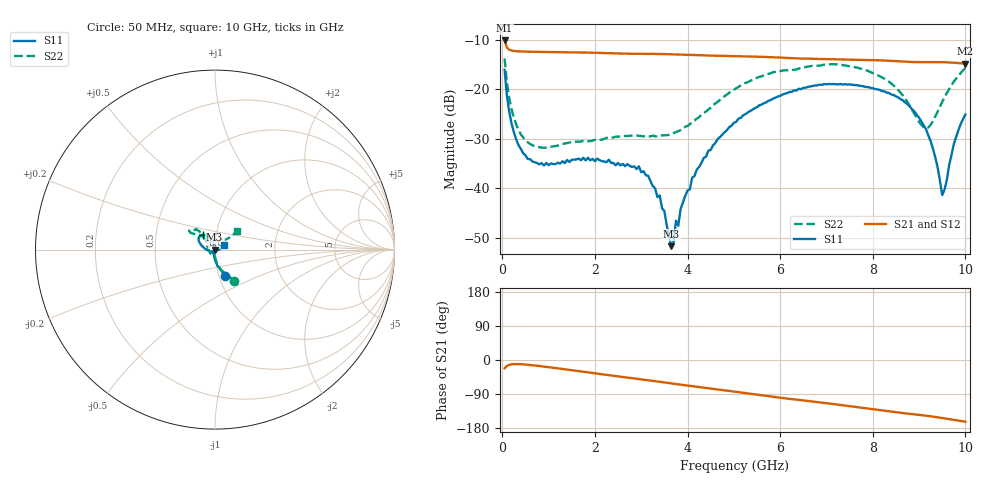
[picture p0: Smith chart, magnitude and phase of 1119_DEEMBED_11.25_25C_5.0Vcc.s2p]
!Hittite Microwave Corp.
!Digital Attenuator/PhaseShifter Rev 1.4.0
!Filename: C:\DATA\DATA\1119_DEEMBED_11.25_25C_5.0Vcc.s2p
!VNA ID: Agilent Technologies,N5224A,MY51441122,A.10.45.03
!Device type:
!2 Port Calibration.
!Temp(C): 25
!Lot Number:
!Serial Number:
!Operator:
!Misc:
!Attenuator:  11.250
# GHZ S DB R 50.0
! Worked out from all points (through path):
!   200 points, 50 MHz to 10 GHz, reference 50 ohm
!   highest |S21| = -10.14 dB at 50 MHz (marker M1); lowest = -14.8 dB at 10 GHz (marker M2)
!   group delay of S21, straight-line fit = 43.4 ps
!   lowest |S11| = -51.7 dB at 3.65 GHz (marker M3), VSWR 1.01, Z = 49.7 + j0.0195 ohm
!   |S11| at or under -10 dB: start of sweep to end of sweep
!   |S22| runs from -31.8 to -13.8 dB; largest |S21 - S12| = 0.00059
!   S11 on the Smith chart (normalised r, x): 50 MHz: 1.07, -0.32; 6.6 GHz: 0.86, +0.14; 10 GHz: 1.10, +0.06
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0.05  -16.07 -69.0  -10.14 -21.6  -10.14 -21.6  -13.79 -58.5
0.1  -21.37 -82.7  -11.60 -15.9  -11.59 -15.9  -18.60 -73.4
0.2  -26.94 -94.5  -12.18 -11.4  -12.18 -11.4  -24.05 -84.2
0.55  -34.11 -115.4  -12.41 -12.5  -12.41 -12.5  -30.71 -95.2
1.75  -33.86 -130.6  -12.58 -30.9  -12.58 -30.9  -30.48 -111.8
2.95  -35.58 -117.8  -12.83 -50.1  -12.84 -50.1  -29.43 -149.0
3.4  -41.48 -131.6  -12.88 -57.5  -12.89 -57.6  -29.43 -170.3
3.65  -51.72 175.7  -12.95 -61.7  -12.96 -61.7  -29.04 176.6
3.7  -50.84 158.6  -12.95 -62.6  -12.96 -62.6  -28.86 173.6
3.75  -46.56 132.4  -12.97 -63.5  -12.97 -63.5  -28.66 171.1
3.8  -47.60 115.8  -12.98 -64.3  -12.98 -64.3  -28.47 167.4
3.85  -44.19 113.9  -13.00 -65.1  -13.01 -65.2  -28.26 164.9
4.1  -37.87 96.9  -13.07 -69.1  -13.08 -69.2  -26.65 152.2
5.05  -26.59 102.7  -13.30 -84.0  -13.32 -84.0  -19.80 129.0
6.6  -19.52 128.8  -13.82 -108.0  -13.84 -108.0  -15.42 139.6
6.7  -19.35 130.5  -13.84 -109.5  -13.85 -109.6  -15.28 140.1
8.35  -20.76 156.9  -14.24 -135.3  -14.24 -135.3  -18.49 137.4
9.15  -28.10 -171.9  -14.50 -147.0  -14.51 -147.0  -27.87 88.3
9.35  -33.79 -149.4  -14.50 -150.3  -14.52 -150.3  -25.49 57.7
9.5  -41.38 -95.2  -14.52 -153.1  -14.54 -153.1  -22.51 45.1
9.75  -31.09 9.7  -14.64 -157.9  -14.65 -157.9  -18.47 39.2
10  -25.12 30.8  -14.83 -162.8  -14.83 -162.8  -15.73 40.0
